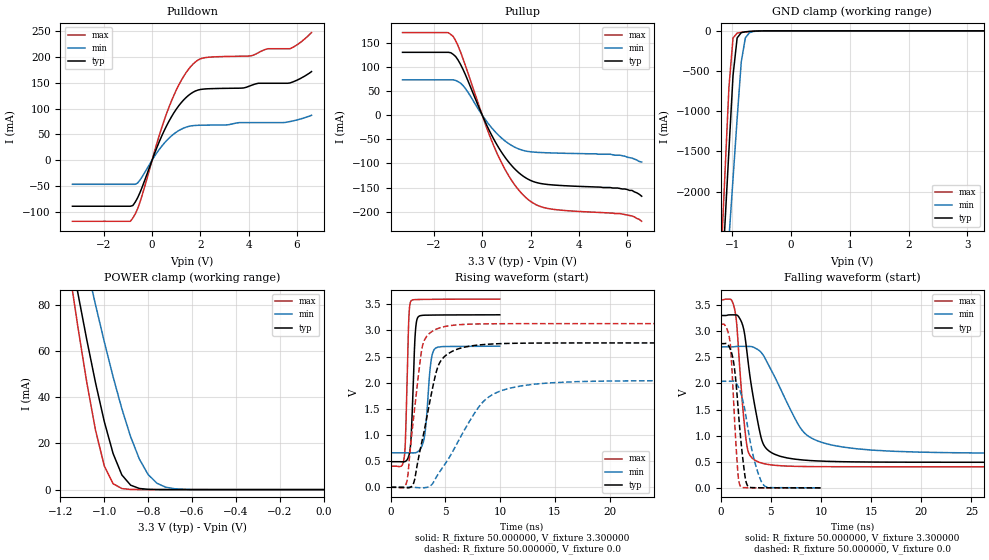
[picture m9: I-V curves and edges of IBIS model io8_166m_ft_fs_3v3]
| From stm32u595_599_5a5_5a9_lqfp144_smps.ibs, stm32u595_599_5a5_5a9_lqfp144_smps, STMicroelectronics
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|   Model io8_166m_ft_fs_3v3
[Model]  io8_166m_ft_fs_3v3
Model_type I/O
Polarity   Non-Inverting
Enable   Active-Low
Vinl =   0.990000V
Vinh =   2.310000V
Vmeas =  1.650000V
Cref =   50.000000pF
Rref =   100.000000M
Vref =   0.0V
C_comp   3.517200pF   3.489400pF   3.557800pF
[Temperature Range]   25.000000   0.140000k   -40.000000
[Pullup Reference]   3.300000V   2.700000V   3.600000V
[Pulldown Reference]   0.0V   0.0V   0.0V
[POWER Clamp Reference]   3.300000V   2.700000V   3.600000V
[GND Clamp Reference]   0.0V   0.0V   0.0V
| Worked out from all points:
|   slope of the pulldown table from 0 to 0.495 V, typ, clamps not added: 8.73 ohm
|   slope of the pullup table from 0 to 0.495 V, typ, clamps not added: 9.64 ohm
|   GND clamp passes 1 mA (typ) near -0.50 V on its own axis
|   POWER clamp passes 1 mA (typ) near -0.85 V on its own axis
|   rising waveform, R_fixture 50.000000, V_fixture 3.300000: 20-80 % time 303ps typ, 460ps min, 244ps max; typ from 0.49 V to 3.3 V
|   rising waveform, R_fixture 50.000000, V_fixture 0.0: 20-80 % time 1.63ns typ, 3.59ns min, 1.01ns max; typ from 0 V to 2.76 V
|   falling waveform, R_fixture 50.000000, V_fixture 3.300000: 20-80 % time 1.39ns typ, 3.34ns min, 786ps max; typ from 3.3 V to 0.49 V
|   falling waveform, R_fixture 50.000000, V_fixture 0.0: 20-80 % time 788ps typ, 1.27ns min, 541ps max; typ from 2.76 V to 0 V
[Pulldown]
|Voltage   I(typ)   I(min)   I(max)
-3.3V     -89.72mA   -47.06mA   -119mA
-900mV    -89.72mA   -47.06mA   -119mA
-500mV    -62.92mA   -38.71mA   -81.44mA
300mV     36.2mA     21.01mA    48.7mA
800mV     84.07mA    46.96mA    114.8mA
1.3V      116.7mA    62.09mA    162.4mA
1.8V      134.4mA    67.39mA    191.2mA
2.3V      138.6mA    67.98mA    199.8mA
4.1V      145.2mA    72.79mA    202.7mA
4.8V      149.4mA    72.79mA    216.5mA
5.7V      149.8mA    74.8mA     216.5mA
6.6V      172mA      87.1mA     247.9mA
[Pullup]
|Voltage   I(typ)   I(min)   I(max)
-3.3V     130.3mA    73.27mA    171.3mA
-1.4V     130.3mA    73.27mA    171mA
-1.2V     126mA      73.27mA    163.1mA
-800mV    95.36mA    61.6mA     117.5mA
100mV     -11.39mA   -7.258mA   -14.51mA
600mV     -60.65mA   -37.83mA   -77.69mA
1.2V      -103.6mA   -62.35mA   -134mA
1.9V      -132.8mA   -75.24mA   -174.9mA
2.7V      -143.6mA   -78mA      -193.3mA
5.6V      -151mA     -83mA      -204mA
6.2V      -156mA     -89mA      -209mA
6.6V      -168mA     -97mA      -220mA
[GND_clamp]
|Voltage   I(typ)   I(min)   I(max)
-3.3V     -9.098A    -9.372A    -9.671A
-1.2V     -3.386A    -4.091A    -2.933A
-1.13V    -2.437A    -3.34A     -1.815A
-1.06V    -1.49A     -2.588A    -705.6mA
-990mV    -555.7mA   -1.839A    -89.03mA
-920mV    -88.12mA   -1.093A    -28.78mA
-850mV    -22.35mA   -387.4mA   -19.84mA
-780mV    -12.12mA   -88.01mA   -13.88mA
-710mV    -7.71mA    -22.52mA   -8.846mA
-640mV    -4.545mA   -7.864mA   -4.87mA
-360mV    -31.12uA   -173.5uA   -8.497uA
3.28V     0A         14.15nA    -7.901nA
[POWER_clamp]
|Voltage   I(typ)   I(min)   I(max)
-3.28V    1.355A     1.167A     1.664A
-1.16V    105.7mA    131.6mA    95.69mA
-1.12V    84.97mA    114mA      70.27mA
-1.08V    65.05mA    96.83mA    46.54mA
-1.04V    46.34mA    80.15mA    25.76mA
-1V       29.51mA    64.13mA    10.3mA
-960mV    15.69mA    48.99mA    2.571mA
-920mV    6.373mA    35.1mA     455.6uA
-840mV    490.7uA    13.24mA    11.36uA
-760mV    27.33uA    2.767mA    278.3nA
-640mV    347.6nA    134.1uA    16.77nA
0V        0A         19.95nA    0A
[Ramp]
| variable   typ   min   max
dV/dt_r  1.65714/1.63206n   1.22460/3.58180n   1.87854/1.00625n
dV/dt_f  1.68606/1.38711n   1.22411/3.33136n   1.91789/0.78141n
R_load = 50.000000
[Rising Waveform]
R_fixture= 50.000000
V_fixture= 3.300000
V_fixture_min= 2.700000
V_fixture_max= 3.600000
|time   V(typ)   V(min)   V(max)
0s        489.9mV    659.8mV    403.5mV
1.261ns   488.6mV    659.8mV    595.8mV
1.662ns   601.2mV    659.6mV    3.199V
1.862ns   910.6mV    659mV      3.564V
2.222ns   2.829V     659.9mV    3.591V
2.503ns   3.255V     683.7mV    3.593V
3.123ns   3.293V     1.006V     3.595V
3.624ns   3.294V     2.294V     3.596V
3.984ns   3.295V     2.635V     3.597V
9.97ns    3.3V       2.7V       3.6V
[Rising Waveform]
R_fixture= 50.000000
V_fixture= 0.0
V_fixture_min= 0.0
V_fixture_max= 0.0
|time   V(typ)   V(min)   V(max)
0s        5.306uV    5.72uV     3.643uV
1.401ns   -9.166mV   40.96uV    53.24mV
1.602ns   -10.69mV   80.54uV    264.9mV
2.102ns   76.88mV    -993uV     1.33V
2.903ns   912.1mV    -9.303mV   2.699V
4.004ns   2.062V     127.7mV    3.008V
4.505ns   2.391V     303.4mV    3.052V
8.408ns   2.729V     1.627V     3.126V
12.01ns   2.757V     1.943V     3.13V
49.85ns   2.762V     2.041V     3.131V
[Falling Waveform]
R_fixture= 50.000000
V_fixture= 3.300000
V_fixture_min= 2.700000
V_fixture_max= 3.600000
|time   V(typ)   V(min)   V(max)
0s        3.3V       2.7V       3.6V
1.401ns   3.312V     2.704V     3.411V
1.602ns   3.31V      2.708V     3.131V
2.202ns   3.107V     2.71V      1.535V
2.703ns   2.463V     2.708V     718.9mV
3.904ns   1.066V     2.618V     485.4mV
4.905ns   693.6mV    2.303V     442.7mV
8.108ns   535.1mV    1.105V     409.7mV
10.91ns   506.6mV    827.6mV    405.1mV
49.85ns   489.9mV    659.8mV    403.5mV
[Falling Waveform]
R_fixture= 50.000000
V_fixture= 0.0
V_fixture_min= 0.0
V_fixture_max= 0.0
|time   V(typ)   V(min)   V(max)
0s        2.762V     2.041V     3.131V
520.5ps   2.766V     2.041V     3.085V
920.9ps   2.673V     2.041V     2.81V
1.301ns   2.389V     2.044V     1.613V
1.682ns   1.657V     1.96V      366.3mV
1.962ns   1.008V     1.836V     32.29mV
2.623ns   60.33mV    1.246V     2.753mV
3.343ns   3.566mV    534.2mV    1.566mV
4.284ns   1.628mV    52.75mV    1.013mV
9.97ns    5.306uV    5.72uV     3.643uV
